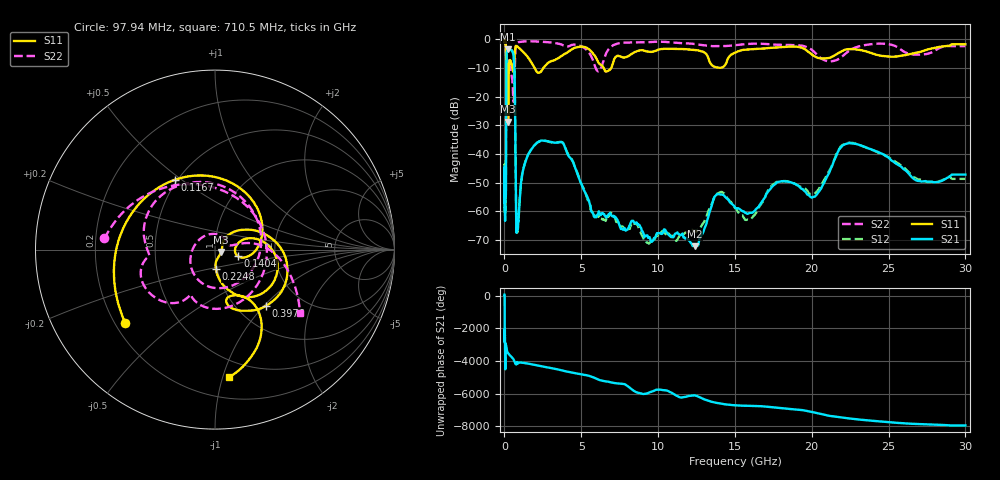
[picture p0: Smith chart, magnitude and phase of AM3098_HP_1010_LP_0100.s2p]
! Date/Time: Thu, Feb 28, 2019 8:41 AM
! Network Analyzer: Agilent Technologies E8364B Rev: A.07.50.67
! Sweep from 0.010 to 30.000 GHz, 1601 Points, Sweep Type: LOG
! Power Supply: 5.022 V, 0.002 A
# Hz S DB R 50
!freq MagS11 AngS11 MagS21 AngS21 MagS12 AngS12 MagS22 AngS22
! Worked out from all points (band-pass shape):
!   1601 points, 10 MHz to 30 GHz, reference 50 ohm
!   highest |S21| = -3.37 dB at 237.5 MHz (marker M1); lowest = -72.2 dB at 12.37 GHz (marker M2)
!   |S21| within 3 dB of the highest: 133 MHz to 606.2 MHz (473.2 MHz wide, 128 % of centre)
!   lowest |S11| = -28.7 dB at 238.7 MHz (marker M3), VSWR 1.08, Z = 53.5 - j1.39 ohm
!   |S11| at or under -10 dB: 199.9 MHz to 290.7 MHz (90.73 MHz wide, 37 % of centre); 1.96 GHz to 2.531 GHz (571.1 MHz wide, 25.4 % of centre); 6.458 GHz to 6.942 GHz (483.8 MHz wide, 7.22 % of centre)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
!   |S22| runs from -21.8 to -0.6 dB; largest |S21 - S12| = 0.01
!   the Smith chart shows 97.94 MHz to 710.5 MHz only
!   S11 on the Smith chart (normalised r, x): 97.94 MHz: 0.24, -0.34; 116.7 MHz: 0.49, +0.47; 140.4 MHz: 1.29, -0.10; 224.8 MHz: 0.99, -0.22; 397.6 MHz: 1.33, -1.02; 710.5 MHz: 0.36, -1.05
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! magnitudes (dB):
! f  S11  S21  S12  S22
! 10 MHz  -0.3  -45.5  -44.2  -0.6
! 38.04 MHz  -0.4  -60.3  -59.6  -0.8
! 97.94 MHz  -3.8  -47.3  -47.4  -4.2
! 116.7 MHz  -7.0  -18.0  -17.9  -10.7
! 140.4 MHz  -17.5  -5.1  -5.1  -10.9
! 144.7 MHz  -19.0  -4.7  -4.7  -10.8
! 184.9 MHz  -8.6  -4.0  -4.0  -7.1
! 224.8 MHz  -19.2  -3.4  -3.4  -8.5
! 237.5 MHz  -28.6  -3.4  -3.3  -8.7
! 238.7 MHz  -28.7  -3.4  -3.3  -8.7
! 397.6 MHz  -7.5  -3.6  -3.6  -9.7
! 550.5 MHz  -11.0  -4.6  -4.6  -18.6
! 649.3 MHz  -6.4  -10.9  -10.9  -14.7
! 710.5 MHz  -2.9  -36.3  -35.9  -4.6
! 762.1 MHz  -2.2  -63.7  -61.3  -2.0
! 833.9 MHz  -2.4  -65.7  -67.4  -1.3
! 2.084 GHz  -11.1  -36.3  -36.2  -0.7
! 3.798 GHz  -5.4  -36.1  -36.0  -2.0
! 7.926 GHz  -6.1  -66.7  -65.7  -1.1
! 12.37 GHz  -3.6  -72.2  -67.0  -1.6
! 22.56 GHz  -3.3  -36.3  -36.1  -3.5
! 30 GHz  -1.7  -47.2  -48.7  -2.3
